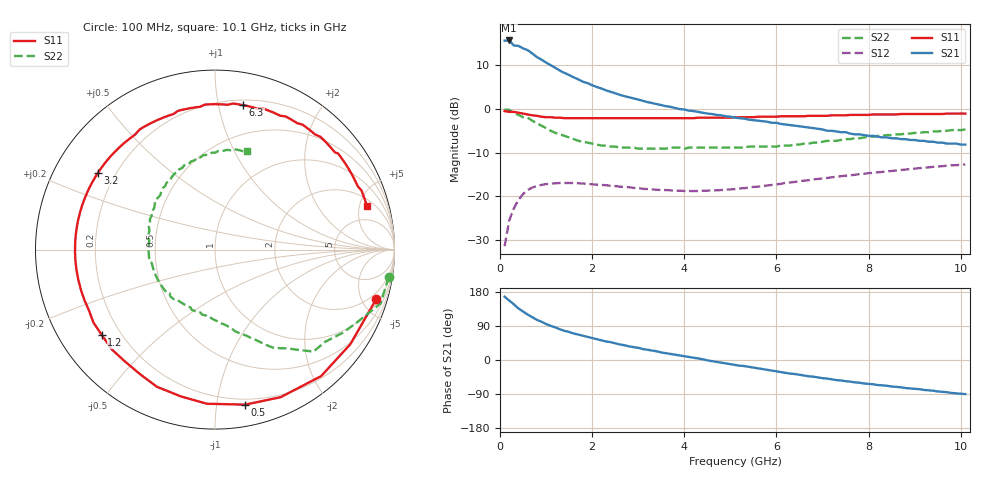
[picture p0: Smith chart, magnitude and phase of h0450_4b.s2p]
!HBFP-0450
!S and NOISE PARAMETERS at Vce=4V  Ic=2mA.  LAST UPDATED  09-04-98
# GHZ S MA R  50
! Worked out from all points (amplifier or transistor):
!   101 points, 100 MHz to 10.1 GHz, reference 50 ohm
!   highest |S21| = 15.6 dB at 200 MHz (marker M1)
!   |S21| within 3 dB of that: start of sweep to 703.8 MHz
!   unconditionally stable (mu >= 1): 3.196 GHz to end of sweep
!   at 1.7 GHz: K = 0.43, MSG = 11.9 dB, |S12| = -17.0 dB
!   at 5.1 GHz: K = 1.44, MAG = 4.2 dB, |S12| = -18.3 dB
!   at 10.1 GHz: K = 1.16, MAG = -0.2 dB, |S12| = -12.7 dB
!   lowest NFmin = 1.49 dB at 1.8 GHz
!   S11 on the Smith chart (normalised r, x): 100 MHz: 1.36, -6.41; 500 MHz: 0.16, -1.20; 1.2 GHz: 0.13, -0.33; 3.2 GHz: 0.13, +0.29; 6.3 GHz: 0.24, +1.18; 10.1 GHz: 2.73, +5.87
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0.1  0.94 -17.0  5.97 167.0  0.027 78.0  0.98 -9.0
0.2  0.92 -35.0  6.01 157.0  0.053 69.0  0.97 -18.0
0.3  0.92 -50.0  5.26 147.0  0.073 60.0  0.89 -27.0
0.4  0.9 -66.0  5.21 136.0  0.091 52.0  0.85 -33.0
0.5  0.88 -79.0  4.88 128.0  0.106 45.0  0.8 -40.0
0.6  0.86 -93.0  4.66 120.0  0.118 39.0  0.79 -46.0
0.8  0.83 -113.0  3.89 106.0  0.131 28.0  0.68 -54.0
1  0.8 -129.0  3.36 95.0  0.138 19.0  0.6 -62.0
1.2  0.79 -143.0  2.93 86.0  0.141 13.0  0.53 -68.0
1.4  0.78 -154.0  2.56 77.0  0.142 8.0  0.49 -73.0
1.6  0.78 -163.0  2.28 70.0  0.142 3.0  0.45 -78.0
1.8  0.78 -172.0  2.03 64.0  0.14 0.0  0.42 -83.0
2.2  0.78 174.0  1.7 52.0  0.135 -6.0  0.38 -94.0
2.6  0.78 162.0  1.44 41.0  0.129 -10.0  0.36 -103.0
3.2  0.78 147.0  1.19 27.0  0.121 -13.0  0.35 -118.0
3.5  0.78 140.0  1.1 20.0  0.118 -14.0  0.35 -125.0
4.5  0.79 118.0  0.88 -1.0  0.116 -13.0  0.36 -148.0
5.1  0.8 105.0  0.79 -13.0  0.121 -13.0  0.36 -163.0
6.3  0.82 79.0  0.65 -36.0  0.144 -16.0  0.38 164.0
6.8  0.83 70.0  0.6 -44.0  0.156 -20.0  0.41 149.0
8.5  0.86 41.0  0.46 -70.0  0.195 -37.0  0.5 107.0
10.1  0.88 16.0  0.39 -90.0  0.231 -58.0  0.58 72.0
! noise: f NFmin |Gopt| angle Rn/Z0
1.8  1.49  0.63  153  0.07
2  1.57  0.62  164  0.05
2.5  1.85  0.65  -178  0.05
3.5  2.24  0.73  -147  0.18
4  2.54  0.76  -134  0.38
5  3.07  0.79  -109  1.09
5.5  3.19  0.83  -98  1.68
7  3.99  0.85  -66  4.22
8  4.35  0.87  -48  6.49
10  5.03  0.87  -17  10.19
